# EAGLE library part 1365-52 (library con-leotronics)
DUAL ROW STRAIGHT HEADER 1364 SERIES. 1.27mm x 1.27mm. Without Fixing Post. SMT Source: http://www.leotronics.co.uk/Conexcon/Data%20Sheets/sec.%20A/1364ing.pdf
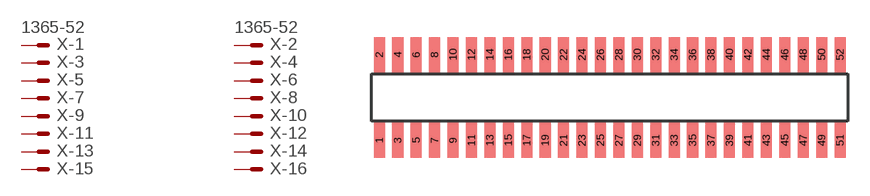
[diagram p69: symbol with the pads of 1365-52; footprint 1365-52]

Designator prefix X; gates -1=MVAL -2=MVAL -3=M -4=M -5=M -6=M -7=M -8=M -9=M -10=M -11=M -12=M -13=M -14=M -15=M -16=M -17=M -18=M -19=M -20=M -21=M -22=M -23=M -24=M -25=M -26=M -27=M -28=M -29=M -30=M -31=M -32=M -33=M -34=M -35=M -36=M -37=M -38=M -39=M -40=M -41=M -42=M -43=M -44=M -45=M -46=M -47=M -48=M -49=M -50=M -51=M -52=M

## 1365-52 (OC_FARNELL: unknown; OC_NEWARK: unknown)  [1365-52]
1  -1:S  pas
2  -2:S  pas
3  -3:S  pas
4  -4:S  pas
5  -5:S  pas
6  -6:S  pas
7  -7:S  pas
8  -8:S  pas
9  -9:S  pas
10  -10:S  pas
11  -11:S  pas
12  -12:S  pas
13  -13:S  pas
14  -14:S  pas
15  -15:S  pas
16  -16:S  pas
17  -17:S  pas
18  -18:S  pas
19  -19:S  pas
20  -20:S  pas
21  -21:S  pas
22  -22:S  pas
23  -23:S  pas
24  -24:S  pas
25  -25:S  pas
26  -26:S  pas
27  -27:S  pas
28  -28:S  pas
29  -29:S  pas
30  -30:S  pas
31  -31:S  pas
32  -32:S  pas
33  -33:S  pas
34  -34:S  pas
35  -35:S  pas
36  -36:S  pas
37  -37:S  pas
38  -38:S  pas
39  -39:S  pas
40  -40:S  pas
41  -41:S  pas
42  -42:S  pas
43  -43:S  pas
44  -44:S  pas
45  -45:S  pas
46  -46:S  pas
47  -47:S  pas
48  -48:S  pas
49  -49:S  pas
50  -50:S  pas
51  -51:S  pas
52  -52:S  pas

## Footprint 1365-52 (pad centres in mm)
DUAL ROW STRAIGHT HEADER 1364 SERIES. 1.27mm x 1.27mm. Without Fixing Post. SMT Source: http://www.leotronics.co.uk/Conexcon/Data%20Sheets/sec.%20A/1364ing.pdf
smd 0.76 x 2.4: 1 -15.875,-2.95; 2 -15.875,2.95; 3 -14.605,-2.95; 4 -14.605,2.95; 5 -13.335,-2.95; 6 -13.335,2.95; 7 -12.065,-2.95; 8 -12.065,2.95; 9 -10.795,-2.95; 10 -10.795,2.95; 11 -9.525,-2.95; 12 -9.525,2.95; 13 -8.255,-2.95; 14 -8.255,2.95; 15 -6.985,-2.95; 16 -6.985,2.95; 17 -5.715,-2.95; 18 -5.715,2.95; 19 -4.445,-2.95; 20 -4.445,2.95; 21 -3.175,-2.95; 22 -3.175,2.95; 23 -1.905,-2.95; 24 -1.905,2.95; 25 -0.635,-2.95; 26 -0.635,2.95; 27 0.635,-2.95; 28 0.635,2.95; 29 1.905,-2.95; 30 1.905,2.95; 31 3.175,-2.95; 32 3.175,2.95; 33 4.445,-2.95; 34 4.445,2.95; 35 5.715,-2.95; 36 5.715,2.95; 37 6.985,-2.95; 38 6.985,2.95; 39 8.255,-2.95; 40 8.255,2.95; 41 9.525,-2.95; 42 9.525,2.95; 43 10.795,-2.95; 44 10.795,2.95; 45 12.065,-2.95; 46 12.065,2.95; 47 13.335,-2.95; 48 13.335,2.95; 49 14.605,-2.95; 50 14.605,2.95; 51 15.875,-2.95; 52 15.875,2.95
